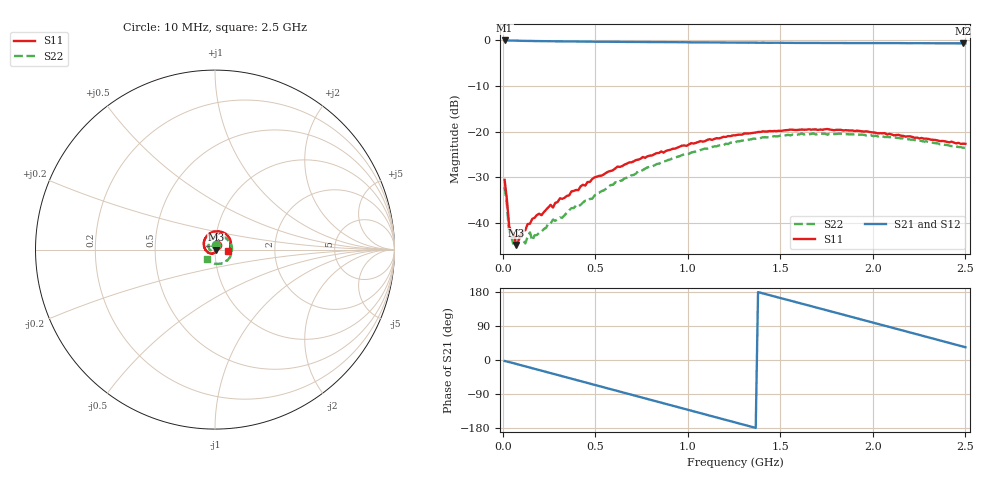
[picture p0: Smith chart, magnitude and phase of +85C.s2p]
!Agilent Technologies,E8364B,MY43040864,A.07.50.48
!Agilent E8364B: A.07.50.48
!Date: Tuesday, September 09, 2025 17:50:17
!Correction: S11(Full 2 Port(1,2))
!S21(Full 2 Port(1,2))
!S12(Full 2 Port(1,2))
!S22(Full 2 Port(1,2))
!S2P File: Measurements: S11, S21, S12, S22:
# Hz S  dB  R 50
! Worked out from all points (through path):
!   201 points, 10 MHz to 2.5 GHz, reference 50 ohm
!   highest |S21| = -0.06 dB at 10 MHz (marker M1); lowest = -0.7 dB at 2.488 GHz (marker M2)
!   group delay of S21, straight-line fit = 361 ps
!   lowest |S11| = -44.7 dB at 72.25 MHz (marker M3), VSWR 1.01, Z = 50.6 - j0.125 ohm
!   |S11| at or under -10 dB: start of sweep to end of sweep
!   |S22| runs from -45.0 to -20.4 dB; largest |S21 - S12| = 0.0044
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1e7  -30.54 68.7  -0.06 -2.6  -0.04 -2.8  -32.12 75.7
2.245e7  -34.85 54.7  -0.06 -4.0  -0.06 -4.1  -35.99 64.4
3.49e7  -40.77 39.5  -0.07 -5.4  -0.06 -5.3  -42.47 41.7
5.98e7  -42.53 14.8  -0.09 -8.6  -0.11 -8.7  -45.03 8.9
7.225e7  -44.74 -12.3  -0.11 -10.2  -0.11 -10.2  -42.71 3.9
9.715e7  -42.59 -22.8  -0.14 -13.5  -0.14 -13.6  -42.57 -14.5
1.2205e8  -41.53 -20.2  -0.14 -16.9  -0.15 -17.0  -44.43 -11.5
1.4695e8  -40.11 -47.4  -0.16 -20.2  -0.17 -20.2  -42.00 -45.6
1.594e8  -39.05 -53.4  -0.18 -21.8  -0.16 -21.8  -43.77 -55.1
2.7145e8  -36.59 -86.8  -0.24 -36.5  -0.24 -36.6  -39.22 -96.8
4.333e8  -31.61 -124.0  -0.30 -57.7  -0.29 -57.7  -35.50 -134.7
6.325e8  -27.70 -156.8  -0.37 -83.6  -0.36 -83.7  -30.80 -179.5
8.4415e8  -24.65 172.5  -0.42 -111.2  -0.41 -111.3  -26.99 140.9
1.06825e9  -22.06 140.1  -0.48 -140.4  -0.48 -140.4  -24.03 104.3
1.255e9  -20.80 114.3  -0.52 -164.6  -0.52 -164.6  -22.35 74.1
1.4791e9  -19.87 86.2  -0.56 166.2  -0.57 166.3  -21.04 39.9
1.6783e9  -19.54 62.5  -0.60 140.7  -0.59 140.6  -20.39 8.1
1.9024e9  -19.86 37.9  -0.61 111.4  -0.64 111.6  -20.55 -26.2
2.08915e9  -20.46 20.3  -0.65 87.2  -0.65 87.3  -21.19 -56.6
2.251e9  -21.47 7.2  -0.67 66.2  -0.64 66.2  -21.96 -83.8
2.48755e9  -22.62 -5.0  -0.69 35.4  -0.68 35.3  -23.51 -127.6
2.5e9  -22.66 -6.1  -0.69 33.7  -0.70 33.8  -23.54 -130.7
